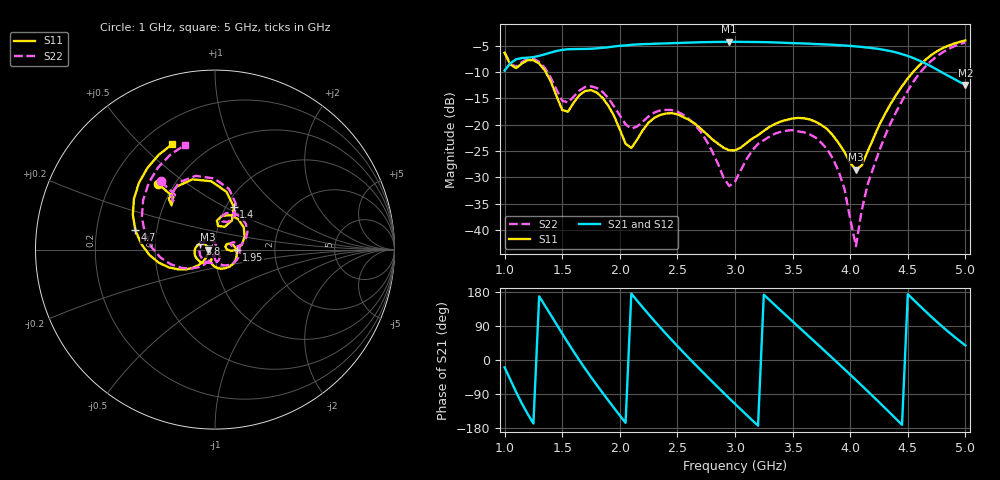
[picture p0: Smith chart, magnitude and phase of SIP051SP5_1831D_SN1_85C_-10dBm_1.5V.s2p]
# GHz  S  dB  R  50
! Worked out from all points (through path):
!   81 points, 1 GHz to 5 GHz, reference 50 ohm
!   highest |S21| = -4.22 dB at 2.95 GHz (marker M1); lowest = -12.4 dB at 5 GHz (marker M2)
!   lowest |S11| = -28.6 dB at 4.05 GHz (marker M3), VSWR 1.08, Z = 46.4 - j0.0993 ohm
!   |S11| at or under -10 dB: 1.358 GHz to 4.545 GHz (3.187 GHz wide, 108 % of centre)
!   |S22| runs from -43.1 to -4.3 dB; largest |S21 - S12| = 0.0036
!   S11 on the Smith chart (normalised r, x): 1 GHz: 0.41, +0.39; 1.4 GHz: 1.09, +0.55; 1.95 GHz: 1.28, -0.00; 3.8 GHz: 0.84, +0.05; 4.7 GHz: 0.38, +0.10; 5 GHz: 0.32, +0.62
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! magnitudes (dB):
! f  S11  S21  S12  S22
! 1 GHz  -6.3  -9.7  -9.7  -6.3
! 1.1 GHz  -9.2  -7.5  -7.5  -9.0
! 1.3 GHz  -8.4  -6.9  -6.9  -8.0
! 1.4 GHz  -11.7  -6.3  -6.3  -11.0
! 1.55 GHz  -17.5  -5.6  -5.6  -15.8
! 1.7 GHz  -13.6  -5.6  -5.6  -12.8
! 1.95 GHz  -18.3  -5.1  -5.1  -16.5
! 2.1 GHz  -24.4  -4.8  -4.8  -20.7
! 2.35 GHz  -18.1  -4.6  -4.5  -17.3
! 2.65 GHz  -19.8  -4.3  -4.3  -20.0
! 2.95 GHz  -24.9  -4.2  -4.2  -31.7
! 3 GHz  -24.9  -4.2  -4.2  -30.8
! 3.15 GHz  -22.6  -4.3  -4.2  -24.9
! 3.3 GHz  -20.4  -4.3  -4.3  -22.3
! 3.7 GHz  -19.4  -4.6  -4.6  -22.4
! 3.8 GHz  -20.8  -4.7  -4.7  -24.6
! 3.95 GHz  -25.2  -4.9  -4.9  -32.2
! 4.05 GHz  -28.6  -5.1  -5.1  -43.1
! 4.15 GHz  -25.2  -5.3  -5.3  -31.5
! 4.35 GHz  -16.1  -6.0  -6.0  -19.8
! 4.7 GHz  -6.8  -8.9  -8.9  -7.9
! 5 GHz  -4.0  -12.4  -12.4  -4.3
